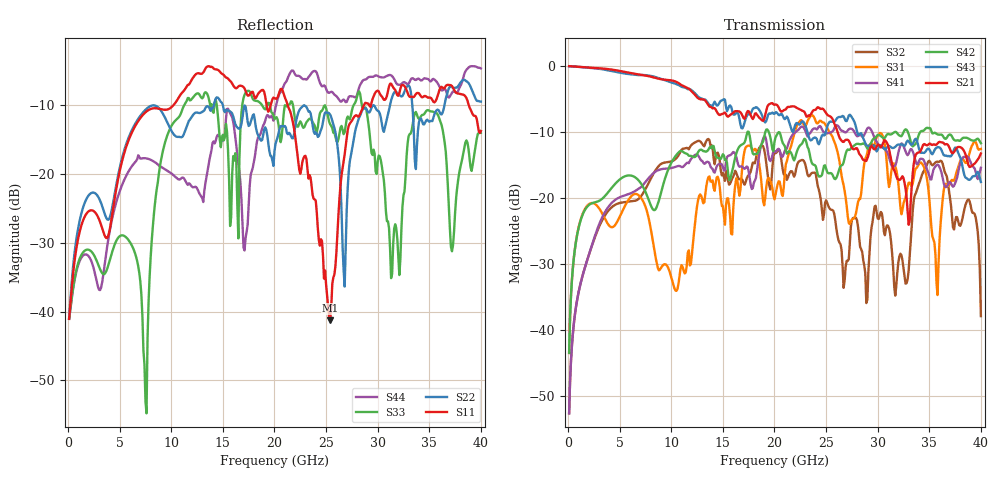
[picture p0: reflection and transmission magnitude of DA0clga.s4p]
! ADC12DJ3200QML-SP
! 196-pin ZMX package
! CLGA Ceramic Package without columns (ceramic land grid array)
! Texas Instruments 4/21/2021
! Single-ended  S-parameters
! PORT#  PORT_NAME  NET_NAME
! PORT1:  DAxN.DIEBUMP DAxN
! PORT2:  DAxN.BGA  DAxN
! PORT3:  DAxP.DIEBUMP DAxP
! PORT4:  DAxP.BGA  DAxP
! Touchstone Ver. 1.0
! Number of ports is 4
# Hz	S	MA	R	50.000000
! SCATTERING PARAMETERS  :
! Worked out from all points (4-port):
!   400 points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, 100 MHz to 40 GHz, reference 50 ohm
!   strongest paths, dB at 100 MHz, 10.1 GHz, 20.1 GHz, 30.1 GHz, 40 GHz:
!     S21: -0.1, -2.3, -5.9, -12.0, -13.3
!     S43: -0.1, -2.6, -7.1, -12.4, -17.6
!     S42: -43.5, -14.4, -10.9, -10.5, -11.7
!     S41: -52.6, -15.5, -13.1, -12.1, -15.5
!     S31: -43.5, -32.6, -19.5, -10.4, -12.6
!     S32: -52.7, -14.5, -13.3, -23.2, -37.9
!   lowest |S11| = -41.3 dB at 25.4 GHz (marker M1), VSWR 1.02, Z = 50.2 + j0.85 ohm
!   |S11| at or under -10 dB: start of sweep to 10.19 GHz; 21.28 GHz to 28.66 GHz (7.375 GHz wide, 29.5 % of centre); 38.84 GHz to end of sweep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
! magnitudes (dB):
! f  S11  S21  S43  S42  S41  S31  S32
! 100 MHz  -41.0  -0.1  -0.1  -43.5  -52.6  -43.5  -52.7
! 7.6 GHz  -10.9  -1.5  -1.5  -19.5  -17.4  -21.8  -18.4
! 9.1 GHz  -10.6  -2.1  -2.1  -18.7  -15.7  -30.4  -14.8
! 13.6 GHz  -4.3  -6.0  -5.8  -12.7  -14.6  -16.9  -11.1
! 25.4 GHz  -41.3  -7.7  -8.5  -16.3  -10.1  -10.2  -21.7
! 28.8 GHz  -9.6  -14.4  -11.7  -12.0  -10.2  -14.1  -31.5
! 40 GHz  -13.7  -13.3  -17.6  -11.7  -15.5  -12.6  -37.9
